| IBIS file stm32g030_031_041_lqfp32.ibs
[IBIS ver]  4.2
[File name] stm32g030_031_041_lqfp32.ibs
[File Rev]  rev1.1
[Date]   01-04-2022
[Source] Data Created at STMicroelectronics
[Notes]  File originated from ELDO simulations.
[Disclaimer]  This information is for modeling purpose only and is
   not guaranted. The information is subject to change without
   notice.
[Copyright] Copyright 2022 STMicroelectronics Inc.
|   Component stm32g030_031_041_lqfp32
[Component] stm32g030_031_041_lqfp32
[Manufacturer] STMicroelectronics
[Package]
| variable   typ   min   max
R_pkg   0.0   0.0   0.0
L_pkg   0.0H   0.0H   0.0H
C_pkg   0.0F   0.0F   0.0F
[Pin]   signal_name   model_name  R_pin L_pin C_pin
1 PB9 io6_i2c_ft 64.896E-3 2.0240E-9 16.235E-15
2 PC14-OSC32_IN io8prog2m25m50m120m_sudq_ft 54.988E-3 1.7405E-9 14.587E-15
3 PC15-OSC32_OUT io8prog2m25m50m120m_sudq_ft 53.017E-3 1.6595E-9 8.197E-15
4 VDD/VDDA POWER 54.033E-3 1.6554E-9 7.363E-15
5 VSS/VSSA GND 56.223E-3 1.7156E-9 10.783E-15
6 PF2-NRST io6reset 61.160E-3 1.8629E-9 10.243E-15
7 PA0 io6_ft 59.987E-3 1.8648E-9 10.852E-15
8 PA1 io6_ft 71.192E-3 2.1932E-9 17.019E-15
9 PA2 io6_ft 71.059E-3 2.1776E-9 16.855E-15
10 PA3 io6_ft 63.005E-3 1.9478E-9 14.439E-15
11 PA4 io6_ft 58.243E-3 1.7981E-9 7.948E-15
12 PA5 io6_ft 55.874E-3 1.7092E-9 8.812E-15
13 PA6 io6_ft 55.141E-3 1.6964E-9 12.212E-15
14 PA7 io6_ft 56.661E-3 1.7554E-9 4.706E-15
15 PB0 io6_ft 61.182E-3 1.8979E-9 13.557E-15
16 PB1 io6_ft 68.639E-3 2.1172E-9 16.500E-15
17 PB2 io6_ft 66.539E-3 2.0692E-9 17.677E-15
18 PA8 io6_ft 71.158E-3 2.1438E-9 11.062E-15
19 PA9 io6_i2c_ft 63.842E-3 1.9327E-9 9.196E-15
20 PC6 io6_ft 58.291E-3 1.7635E-9 11.677E-15
21 PA10 io6_i2c_ft 54.700E-3 1.6700E-9 6.891E-15
22 PA11 io6_i2c_ft 53.046E-3 1.6525E-9 10.905E-15
23 PA12 io6_i2c_ft 62.866E-3 1.9450E-9 11.111E-15
24 PA13 io6_ft 75.711E-3 2.3060E-9 17.278E-15
25 PA14-BOOT0 io6_ft 74.224E-3 2.2583E-9 19.736E-15
26 PA15 io6_ft 65.224E-3 2.0006E-9 8.439E-15
27 PB3 io6_ft 59.281E-3 1.8183E-9 10.281E-15
28 PB4 io6_ft 56.029E-3 1.7169E-9 8.461E-15
29 PB5 io6_ft 55.139E-3 1.6969E-9 12.383E-15
30 PB6 io6_i2c_ft 56.372E-3 1.7463E-9 4.202E-15
31 PB7 io6_i2c_ft 59.845E-3 1.8672E-9 13.676E-15
32 PB8 io6_i2c_ft 66.777E-3 2.0705E-9 14.725E-15
[Model Selector] io8prog2m25m50m120m_sudq_ft
iols8p_sudq_ft_pd_lv  "IO low speed, PD=40kOhm - 1P8V"
iols8p_sudq_ft_pu_lv  "IO low speed, PU=40kOhm - 1P8V"
iols8p_sudq_ft_lv  "IO low speed - 1P8V"
iols8p_sudq_ft_pd  "IO low speed, PD=40kOhm - 3P3V"
iols8p_sudq_ft_pu  "IO low speed, PU=40kOhm - 3P3V"
iols8p_sudq_ft  "IO low speed - 3P3V"
iofs8p_sudq_ft_pd_lv  "IO full speed, PD=40kOhm - 1P8V"
iofs8p_sudq_ft_pu_lv  "IO full speed, PU=40kOhm - 1P8V"
iofs8p_sudq_ft_lv  "IO full speed - 1P8V"
iofs8p_sudq_ft_pd  "IO full speed, PD=40kOhm - 3P3V"
iofs8p_sudq_ft_pu  "IO full speed, PU=40kOhm - 3P3V"
iofs8p_sudq_ft  "IO full speed - 3P3V"
ioms8p_sudq_ft_pd_lv  "IO medium speed, PD=40kOhm - 1P8V"
ioms8p_sudq_ft_pu_lv  "IO medium speed, PU=40kOhm - 1P8V"
ioms8p_sudq_ft_lv  "IO medium speed - 1P8V"
ioms8p_sudq_ft_pd  "IO medium speed, PD=40kOhm - 3P3V"
ioms8p_sudq_ft_pu  "IO medium speed, PU=40kOhm - 3P3V"
ioms8p_sudq_ft  "IO medium speed - 3P3V"
iohs8p_sudq_ft_pd_lv  "IO high speed, PD=40kOhm - 1P8V"
iohs8p_sudq_ft_pu_lv  "IO high speed, PU=40kOhm - 1P8V"
iohs8p_sudq_ft_lv  "IO high speed - 1P8V"
iohs8p_sudq_ft_pd  "IO high speed, PD=40kOhm - 3P3V"
iohs8p_sudq_ft_pu  "IO high speed, PU=40kOhm - 3P3V"
iohs8p_sudq_ft  "IO high speed - 3P3V"
[Model Selector] io6_ft
io6_ft_1v8_highspeed_pd  "GPIO-1.8V range - high speed - pull down"
io6_ft_1v8_fastspeed_pd  "GPIO-1.8V range - fast speed - pull down"
io6_ft_1v8_mediumspeed_pd  "GPIO-1.8V range - medium speed - pull down"
io6_ft_1v8_lowspeed_pd  "GPIO-1.8V range - low speed - pull down"
io6_ft_1v8_highspeed_pu  "GPIO-1.8V range - high speed - pull up"
io6_ft_1v8_fastspeed_pu  "GPIO-1.8V range - fast speed - pull up"
io6_ft_1v8_mediumspeed_pu  "GPIO-1.8V range - medium speed - pull up"
io6_ft_1v8_lowspeed_pu  "GPIO-1.8V range - low speed - pull up"
io6_ft_1v8_highspeed  "GPIO-1.8V range - high speed"
io6_ft_1v8_fastspeed  "GPIO-1.8V range - fast speed"
io6_ft_1v8_mediumspeed  "GPIO-1.8V range - medium speed"
io6_ft_1v8_lowspeed  "GPIO-1.8V range - low speed"
io6_ft_3v3_highspeed_pd  "GPIO-3.3V range - high speed - pull down"
io6_ft_3v3_fastspeed_pd  "GPIO-3.3V range - fast speed - pull down"
io6_ft_3v3_mediumspeed_pd  "GPIO-3.3V range - medium speed - pull down"
io6_ft_3v3_lowspeed_pd  "GPIO-3.3V range - low speed - pull down"
io6_ft_3v3_highspeed_pu  "GPIO-3.3V range - high speed - pull up"
io6_ft_3v3_fastspeed_pu  "GPIO-3.3V range - fast speed - pull up"
io6_ft_3v3_mediumspeed_pu  "GPIO-3.3V range - medium speed - pull up"
io6_ft_3v3_lowspeed_pu  "GPIO-3.3V range - low speed - pull up"
io6_ft_3v3_highspeed  "GPIO-3.3V range - high speed"
io6_ft_3v3_fastspeed  "GPIO-3.3V range - fast speed"
io6_ft_3v3_mediumspeed  "GPIO-3.3V range - medium speed"
io6_ft_3v3_lowspeed  "GPIO-3.3V range - low speed"
[Model Selector] io6_i2c_ft
io6_ft_1v8_highspeed_pd  "GPIO-1.8V range - high speed - pull down"
io6_ft_1v8_fastspeed_pd  "GPIO-1.8V range - fast speed - pull down"
io6_ft_1v8_mediumspeed_pd  "GPIO-1.8V range - medium speed - pull down"
io6_ft_1v8_lowspeed_pd  "GPIO-1.8V range - low speed - pull down"
io6_ft_1v8_highspeed_pu  "GPIO-1.8V range - high speed - pull up"
io6_ft_1v8_fastspeed_pu  "GPIO-1.8V range - fast speed - pull up"
io6_ft_1v8_mediumspeed_pu  "GPIO-1.8V range - medium speed - pull up"
io6_ft_1v8_lowspeed_pu  "GPIO-1.8V range - low speed - pull up"
io6_ft_1v8_highspeed  "GPIO-1.8V range - high speed"
io6_ft_1v8_fastspeed  "GPIO-1.8V range - fast speed"
io6_ft_1v8_mediumspeed  "GPIO-1.8V range - medium speed"
io6_ft_1v8_lowspeed  "GPIO-1.8V range - low speed"
io6_ft_3v3_highspeed_pd  "GPIO-3.3V range - high speed - pull down"
io6_ft_3v3_fastspeed_pd  "GPIO-3.3V range - fast speed - pull down"
io6_ft_3v3_mediumspeed_pd  "GPIO-3.3V range - medium speed - pull down"
io6_ft_3v3_lowspeed_pd  "GPIO-3.3V range - low speed - pull down"
io6_ft_3v3_highspeed_pu  "GPIO-3.3V range - high speed - pull up"
io6_ft_3v3_fastspeed_pu  "GPIO-3.3V range - fast speed - pull up"
io6_ft_3v3_mediumspeed_pu  "GPIO-3.3V range - medium speed - pull up"
io6_ft_3v3_lowspeed_pu  "GPIO-3.3V range - low speed - pull up"
io6_ft_3v3_highspeed  "GPIO-3.3V range - high speed"
io6_ft_3v3_fastspeed  "GPIO-3.3V range - fast speed"
io6_ft_3v3_mediumspeed  "GPIO-3.3V range - medium speed"
io6_ft_3v3_lowspeed  "GPIO-3.3V range - low speed"
io6_ft_1v8_highi2c_pd   "GPIO-1.8V range - high   speed i2c mode - pd"
io6_ft_1v8_fasti2c_pd   "GPIO-1.8V range - fast   speed i2c mode - pd"
io6_ft_1v8_mediumi2c_pd  "GPIO-1.8V range - medium speed i2c mode - pd"
io6_ft_1v8_lowi2c_pd   "GPIO-1.8V range - low   speed i2c mode - pd"
io6_ft_1v8_highi2c_pu   "GPIO-1.8V range - high   speed i2c mode - pu"
io6_ft_1v8_fasti2c_pu   "GPIO-1.8V range - fast   speed i2c mode - pu"
io6_ft_1v8_mediumi2c_pu  "GPIO-1.8V range - medium speed i2c mode - pu"
io6_ft_1v8_lowi2c_pu   "GPIO-1.8V range - low   speed i2c mode - pu"
io6_ft_1v8_highi2c   "GPIO-1.8V range - high   speed i2c mode"
io6_ft_1v8_fasti2c   "GPIO-1.8V range - fast   speed i2c mode"
io6_ft_1v8_mediumi2c   "GPIO-1.8V range - medium speed i2c mode"
io6_ft_1v8_lowi2c   "GPIO-1.8V range - low   speed i2c mode"
io6_ft_3v3_highi2c_pd   "GPIO-3.3V range - high   speed i2c mode - pd"
io6_ft_3v3_fasti2c_pd   "GPIO-3.3V range - fast   speed i2c mode - pd"
io6_ft_3v3_mediumi2c_pd  "GPIO-3.3V range - medium speed i2c mode - pd"
io6_ft_3v3_lowi2c_pd   "GPIO-3.3V range - low   speed i2c mode - pd"
io6_ft_3v3_highi2c_pu   "GPIO-3.3V range - high   speed i2c mode - pu"
io6_ft_3v3_fasti2c_pu   "GPIO-3.3V range - fast   speed i2c mode - pu"
io6_ft_3v3_mediumi2c_pu  "GPIO-3.3V range - medium speed i2c mode - pu"
io6_ft_3v3_lowi2c_pu   "GPIO-3.3V range - low   speed i2c mode - pu"
io6_ft_3v3_highi2c   "GPIO-3.3V range - high   speed i2c mode"
io6_ft_3v3_fasti2c   "GPIO-3.3V range - fast   speed i2c mode"
io6_ft_3v3_mediumi2c   "GPIO-3.3V range - medium speed i2c mode"
io6_ft_3v3_lowi2c   "GPIO-3.3V range - low   speed i2c mode"
io6_i2c_ft_1v8_pd  "GPIO-1.8V I2C fm+ - pd"
io6_i2c_ft_3v3_pd  "GPIO-3.3V I2C fm+ - pd"
io6_i2c_ft_1v8_pu  "GPIO-1.8V I2C fm+ - pu"
io6_i2c_ft_3v3_pu  "GPIO-3.3V I2C fm+ - pu"
io6_i2c_ft_1v8   "GPIO-1.8V I2C fm+"
io6_i2c_ft_3v3   "GPIO-3.3V I2C fm+"
[Model Selector] io6reset
io6_ft_1v8_highspeed_pd  "GPIO-1.8V range - high speed - pull down"
io6_ft_1v8_fastspeed_pd  "GPIO-1.8V range - fast speed - pull down"
io6_ft_1v8_mediumspeed_pd  "GPIO-1.8V range - medium speed - pull down"
io6_ft_1v8_lowspeed_pd  "GPIO-1.8V range - low speed - pull down"
io6_ft_1v8_highspeed_pu  "GPIO-1.8V range - high speed - pull up"
io6_ft_1v8_fastspeed_pu  "GPIO-1.8V range - fast speed - pull up"
io6_ft_1v8_mediumspeed_pu  "GPIO-1.8V range - medium speed - pull up"
io6_ft_1v8_lowspeed_pu  "GPIO-1.8V range - low speed - pull up"
io6_ft_1v8_highspeed  "GPIO-1.8V range - high speed"
io6_ft_1v8_fastspeed  "GPIO-1.8V range - fast speed"
io6_ft_1v8_mediumspeed  "GPIO-1.8V range - medium speed"
io6_ft_1v8_lowspeed  "GPIO-1.8V range - low speed"
io6_ft_3v3_highspeed_pd  "GPIO-3.3V range - high speed - pull down"
io6_ft_3v3_fastspeed_pd  "GPIO-3.3V range - fast speed - pull down"
io6_ft_3v3_mediumspeed_pd  "GPIO-3.3V range - medium speed - pull down"
io6_ft_3v3_lowspeed_pd  "GPIO-3.3V range - low speed - pull down"
io6_ft_3v3_highspeed_pu  "GPIO-3.3V range - high speed - pull up"
io6_ft_3v3_fastspeed_pu  "GPIO-3.3V range - fast speed - pull up"
io6_ft_3v3_mediumspeed_pu  "GPIO-3.3V range - medium speed - pull up"
io6_ft_3v3_lowspeed_pu  "GPIO-3.3V range - low speed - pull up"
io6_ft_3v3_highspeed  "GPIO-3.3V range - high speed"
io6_ft_3v3_fastspeed  "GPIO-3.3V range - fast speed"
io6_ft_3v3_mediumspeed  "GPIO-3.3V range - medium speed"
io6_ft_3v3_lowspeed  "GPIO-3.3V range - low speed"
ioreset_1v2_pu  "RESET 1.2V range with PU"
ioreset_1v2  "RESET 1.2V range"
ioreset_1v8_pu  "RESET 1.8V range with PU"
ioreset_1v8  "RESET 1.8V range"
ioreset_3v3_pu  "RESET 3.3V range with PU"
ioreset_3v3  "RESET 3.3V range"
| Models and submodels in the file (84): iols8p_sudq_ft_pd_lv (I/O), iols8p_sudq_ft_pu_lv (I/O), iols8p_sudq_ft_lv (I/O), iols8p_sudq_ft_pd (I/O), iols8p_sudq_ft_pu (I/O), iols8p_sudq_ft (I/O), iofs8p_sudq_ft_pd_lv (I/O), iofs8p_sudq_ft_pu_lv (I/O), iofs8p_sudq_ft_lv (I/O), iofs8p_sudq_ft_pd (I/O), iofs8p_sudq_ft_pu (I/O), iofs8p_sudq_ft (I/O), ioms8p_sudq_ft_pd_lv (I/O), ioms8p_sudq_ft_pu_lv (I/O), ioms8p_sudq_ft_lv (I/O), ioms8p_sudq_ft_pd (I/O), ioms8p_sudq_ft_pu (I/O), ioms8p_sudq_ft (I/O), iohs8p_sudq_ft_pd_lv (I/O), iohs8p_sudq_ft_pu_lv (I/O), iohs8p_sudq_ft_lv (I/O), iohs8p_sudq_ft_pd (I/O), iohs8p_sudq_ft_pu (I/O), iohs8p_sudq_ft (I/O), io6_ft_1v8_highspeed_pd (I/O), io6_ft_1v8_fastspeed_pd (I/O), io6_ft_1v8_mediumspeed_pd (I/O), io6_ft_1v8_lowspeed_pd (I/O), io6_ft_1v8_highspeed_pu (I/O), io6_ft_1v8_fastspeed_pu (I/O), io6_ft_1v8_mediumspeed_pu (I/O), io6_ft_1v8_lowspeed_pu (I/O), io6_ft_1v8_highspeed (I/O), io6_ft_1v8_fastspeed (I/O), io6_ft_1v8_mediumspeed (I/O), io6_ft_1v8_lowspeed (I/O), io6_ft_3v3_highspeed_pd (I/O), io6_ft_3v3_fastspeed_pd (I/O), io6_ft_3v3_mediumspeed_pd (I/O), io6_ft_3v3_lowspeed_pd (I/O), io6_ft_3v3_highspeed_pu (I/O), io6_ft_3v3_fastspeed_pu (I/O), io6_ft_3v3_mediumspeed_pu (I/O), io6_ft_3v3_lowspeed_pu (I/O), io6_ft_3v3_highspeed (I/O), io6_ft_3v3_fastspeed (I/O), io6_ft_3v3_mediumspeed (I/O), io6_ft_3v3_lowspeed (I/O), io6_i2c_ft_1v8_pd (I/O_open_drain), io6_i2c_ft_3v3_pd (I/O_open_drain), io6_i2c_ft_1v8_pu (I/O_open_drain), io6_i2c_ft_3v3_pu (I/O_open_drain), io6_i2c_ft_1v8 (I/O_open_drain), io6_i2c_ft_3v3 (I/O_open_drain), io6_ft_1v8_highi2c_pd (I/O_open_drain), io6_ft_1v8_fasti2c_pd (I/O_open_drain), io6_ft_1v8_mediumi2c_pd (I/O_open_drain), io6_ft_1v8_lowi2c_pd (I/O_open_drain), io6_ft_1v8_highi2c_pu (I/O_open_drain), io6_ft_1v8_fasti2c_pu (I/O_open_drain), io6_ft_1v8_mediumi2c_pu (I/O_open_drain), io6_ft_1v8_lowi2c_pu (I/O_open_drain), io6_ft_1v8_highi2c (I/O_open_drain), io6_ft_1v8_fasti2c (I/O_open_drain), io6_ft_1v8_mediumi2c (I/O_open_drain), io6_ft_1v8_lowi2c (I/O_open_drain), io6_ft_3v3_highi2c_pd (I/O_open_drain), io6_ft_3v3_fasti2c_pd (I/O_open_drain), io6_ft_3v3_mediumi2c_pd (I/O_open_drain), io6_ft_3v3_lowi2c_pd (I/O_open_drain), io6_ft_3v3_highi2c_pu (I/O_open_drain), io6_ft_3v3_fasti2c_pu (I/O_open_drain), io6_ft_3v3_mediumi2c_pu (I/O_open_drain), io6_ft_3v3_lowi2c_pu (I/O_open_drain), io6_ft_3v3_highi2c (I/O_open_drain), io6_ft_3v3_fasti2c (I/O_open_drain), io6_ft_3v3_mediumi2c (I/O_open_drain), io6_ft_3v3_lowi2c (I/O_open_drain), ioreset_1v2_pu (I/O_open_drain), ioreset_1v2 (I/O_open_drain)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
